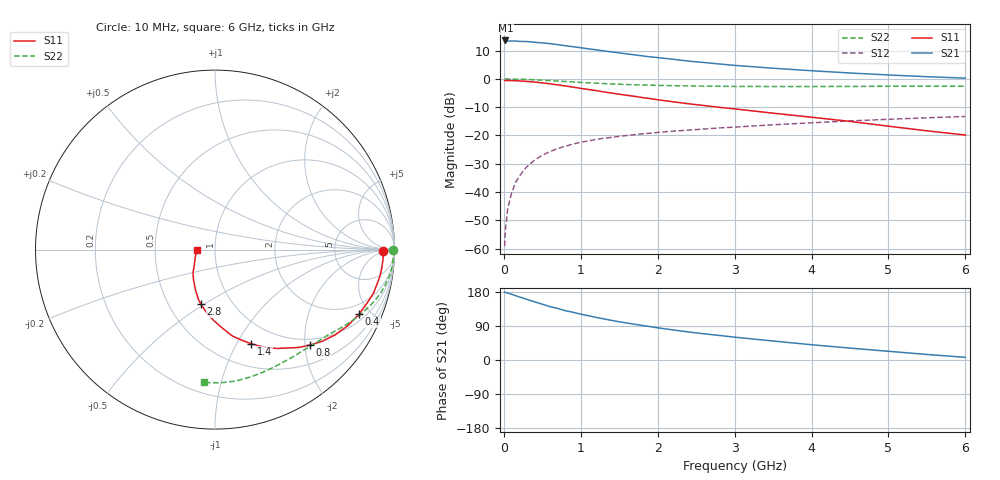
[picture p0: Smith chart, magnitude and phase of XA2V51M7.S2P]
! SIEMENS Discrete & RF Semiconductors
! BFY180
! Si NPN RF Bipolar Junction Transistor in MICRO-X
! VCE = 2.5 V  IC = 1.7 mA
! Common Emitter S-Parameters:  May  1997
# GHz  S  MA  R  50
!  f  S11  S21  S12  S22
! GHz  MAG  ANG  MAG  ANG  MAG  ANG  MAG  ANG
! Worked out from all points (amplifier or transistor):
!   36 points, 10 MHz to 6 GHz, reference 50 ohm
!   highest |S21| = 13.6 dB at 20 MHz (marker M1)
!   |S21| within 3 dB of that: start of sweep to 1.107 GHz
!   unconditionally stable (mu >= 1): 2.895 GHz to end of sweep
!   at 250 MHz: K = 0.11, MSG = 22.9 dB, |S12| = -32.7 dB
!   at 1.4 GHz: K = 0.66, MSG = 15.1 dB, |S12| = -20.7 dB
!   at 6 GHz: K = 1.08, MAG = 5.1 dB, |S12| = -13.3 dB
!   S11 on the Smith chart (normalised r, x): 10 MHz: 29, -5; 400 MHz: 1.34, -4.27; 800 MHz: 0.87, -2.10; 1.4 GHz: 0.75, -1.15; 2.8 GHz: 0.72, -0.49; 6 GHz: 0.82, -0.01
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0.01  0.9353 -0.6  4.68 179.3  0.0011 91.8  0.9942 -0.2
0.02  0.9339 -1.2  4.792 178.4  0.0021 90.8  0.9999 -0.7
0.05  0.9382 -2.9  4.676 176.7  0.005 89.2  0.9969 -1.6
0.1  0.9353 -6.4  4.688 173.5  0.0095 88.2  0.9927 -3.2
0.15  0.93 -9.5  4.687 170.0  0.0145 83.5  0.9937 -4.9
0.3  0.9015 -18.6  4.59 159.8  0.0281 78.2  0.9779 -9.4
0.4  0.8798 -24.2  4.446 153.5  0.0366 74.8  0.9668 -12.3
0.6  0.8205 -35.4  4.21 140.8  0.0519 67.9  0.9357 -17.6
0.8  0.7489 -45.3  3.867 130.2  0.0647 62.2  0.9001 -22.3
1  0.6806 -53.6  3.561 121.1  0.0759 57.0  0.8687 -26.4
1.1  0.6503 -57.9  3.402 116.8  0.0801 55.0  0.8542 -28.1
1.2  0.6211 -61.6  3.274 112.4  0.085 53.1  0.8412 -29.9
1.4  0.5626 -68.9  3.004 104.5  0.0925 50.0  0.8153 -33.2
1.6  0.5132 -75.3  2.77 97.6  0.0999 47.7  0.7965 -36.1
1.8  0.4677 -81.2  2.555 91.2  0.1068 45.6  0.781 -38.9
2.2  0.3944 -91.1  2.227 79.3  0.119 41.6  0.7596 -44.4
2.6  0.3389 -99.9  1.955 69.1  0.1298 38.7  0.7449 -49.5
2.8  0.3147 -104.3  1.838 64.9  0.136 37.2  0.7413 -52.0
3.5  0.2478 -116.2  1.545 50.1  0.1543 32.4  0.7331 -60.8
4.5  0.1772 -133.8  1.273 31.4  0.1807 25.2  0.7364 -73.9
5.5  0.1207 -156.7  1.096 14.6  0.2053 17.7  0.7431 -87.8
6  0.1018 -177.4  1.032 7.1  0.2166 13.4  0.7427 -94.9
